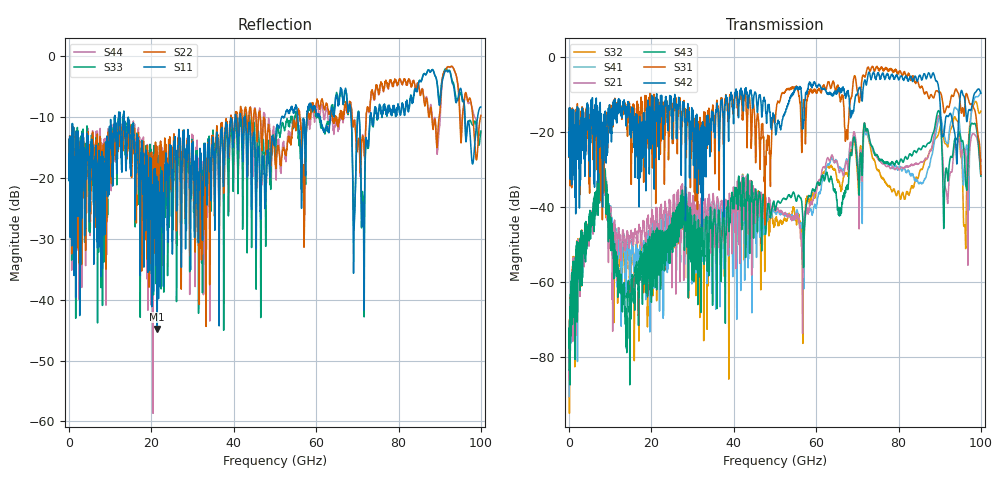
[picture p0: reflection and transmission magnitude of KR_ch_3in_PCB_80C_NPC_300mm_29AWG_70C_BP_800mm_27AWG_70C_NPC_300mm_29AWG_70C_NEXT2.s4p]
# GHz S RI R 45
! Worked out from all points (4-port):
!   4000 points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, 25 MHz to 100 GHz, reference 45 ohm
!   strongest paths, dB at 25 MHz, 25.02 GHz, 50.02 GHz, 75.03 GHz, 100 GHz:
!     S42: -20.0, -17.9, -18.0, -4.4, -9.7
!     S31: -20.0, -13.7, -17.3, -3.0, -31.3
!     S43: -83.4, -44.5, -40.7, -26.6, -31.8
!     S21: -82.5, -46.5, -40.8, -27.3, -27.3
!     S41: -90.4, -50.0, -41.1, -27.0, -9.7
!     S32: -84.5, -44.2, -43.9, -30.2, -14.5
!   lowest |S11| = -44.8 dB at 21.43 GHz (marker M1), VSWR 1.01, Z = 44.5 - j0.0596 ohm
!   |S11| at or under -10 dB: start of sweep to 11.05 GHz; 13.38 GHz to 40.37 GHz (26.99 GHz wide, 100 % of centre); 42.8 GHz to 51.67 GHz (8.863 GHz wide, 18.8 % of centre)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
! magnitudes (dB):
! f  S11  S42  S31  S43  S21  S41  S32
! 25 MHz  -16.0  -20.0  -20.0  -83.4  -82.5  -90.4  -84.5
! 8.025 GHz  -17.9  -24.5  -24.7  -24.8  -25.9  -25.3  -25.7
! 13.62 GHz  -13.2  -14.9  -14.0  -68.3  -50.1  -56.0  -56.1
! 21.43 GHz  -44.8  -16.6  -19.9  -45.6  -40.3  -43.2  -47.9
! 71.95 GHz  -15.7  -6.6  -5.1  -18.8  -19.3  -20.1  -18.8
! 96.1 GHz  -9.6  -11.6  -13.3  -28.6  -24.7  -27.3  -44.9
! 100 GHz  -8.3  -9.7  -31.3  -31.8  -27.3  -9.7  -14.5
